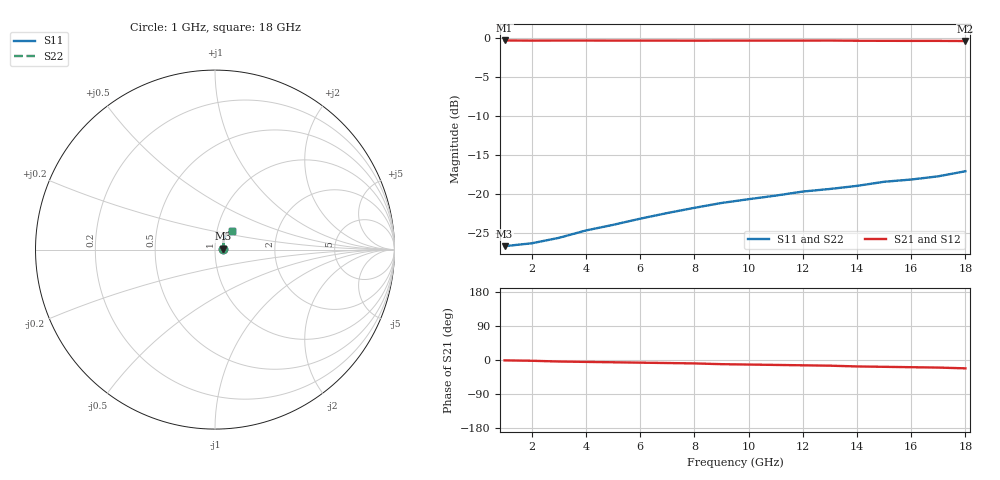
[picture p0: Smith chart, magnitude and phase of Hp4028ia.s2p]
!HPND-4028 beam lead PIN diode
!Series configuration S-parameters If=1 mA.  Last updated 10/3/97
# mhz s ma r 50
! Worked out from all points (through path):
!   18 points, 1 GHz to 18 GHz, reference 50 ohm
!   highest |S21| = -0.37 dB at 1 GHz (marker M1); lowest = -0.4 dB at 18 GHz (marker M2)
!   group delay of S21, straight-line fit = 3.33 ps
!   lowest |S11| = -26.7 dB at 1 GHz (marker M3), VSWR 1.10, Z = 54.8 + j0.616 ohm
!   |S11| at or under -10 dB: start of sweep to end of sweep
!   |S22| runs from -26.7 to -17.1 dB; largest |S21 - S12| = 0
1000  0.046 7.0  0.958 -1.0  0.958 -1.0  0.046 7.0
2000  0.048 20.0  0.956 -2.0  0.956 -2.0  0.048 20.0
3000  0.052 29.0  0.957 -4.0  0.957 -4.0  0.052 29.0
4000  0.058 36.0  0.957 -5.0  0.957 -5.0  0.058 36.0
5000  0.063 42.0  0.956 -6.0  0.956 -6.0  0.063 42.0
6000  0.069 46.0  0.956 -7.0  0.956 -7.0  0.069 46.0
7000  0.075 48.0  0.956 -8.0  0.956 -8.0  0.075 48.0
8000  0.081 50.0  0.955 -9.0  0.955 -9.0  0.081 50.0
9000  0.087 51.0  0.956 -11.0  0.956 -11.0  0.087 51.0
10000  0.092 52.0  0.956 -12.0  0.956 -12.0  0.092 52.0
11000  0.097 53.0  0.956 -13.0  0.956 -13.0  0.097 53.0
12000  0.103 52.0  0.956 -14.0  0.956 -14.0  0.103 52.0
13000  0.107 51.0  0.957 -15.0  0.957 -15.0  0.107 51.0
14000  0.112 51.0  0.954 -17.0  0.954 -17.0  0.112 51.0
15000  0.119 51.0  0.953 -18.0  0.953 -18.0  0.119 51.0
16000  0.123 51.0  0.952 -19.0  0.952 -19.0  0.123 51.0
17000  0.129 49.0  0.952 -20.0  0.952 -20.0  0.129 49.0
18000  0.139 48.0  0.95 -22.0  0.95 -22.0  0.139 48.0
